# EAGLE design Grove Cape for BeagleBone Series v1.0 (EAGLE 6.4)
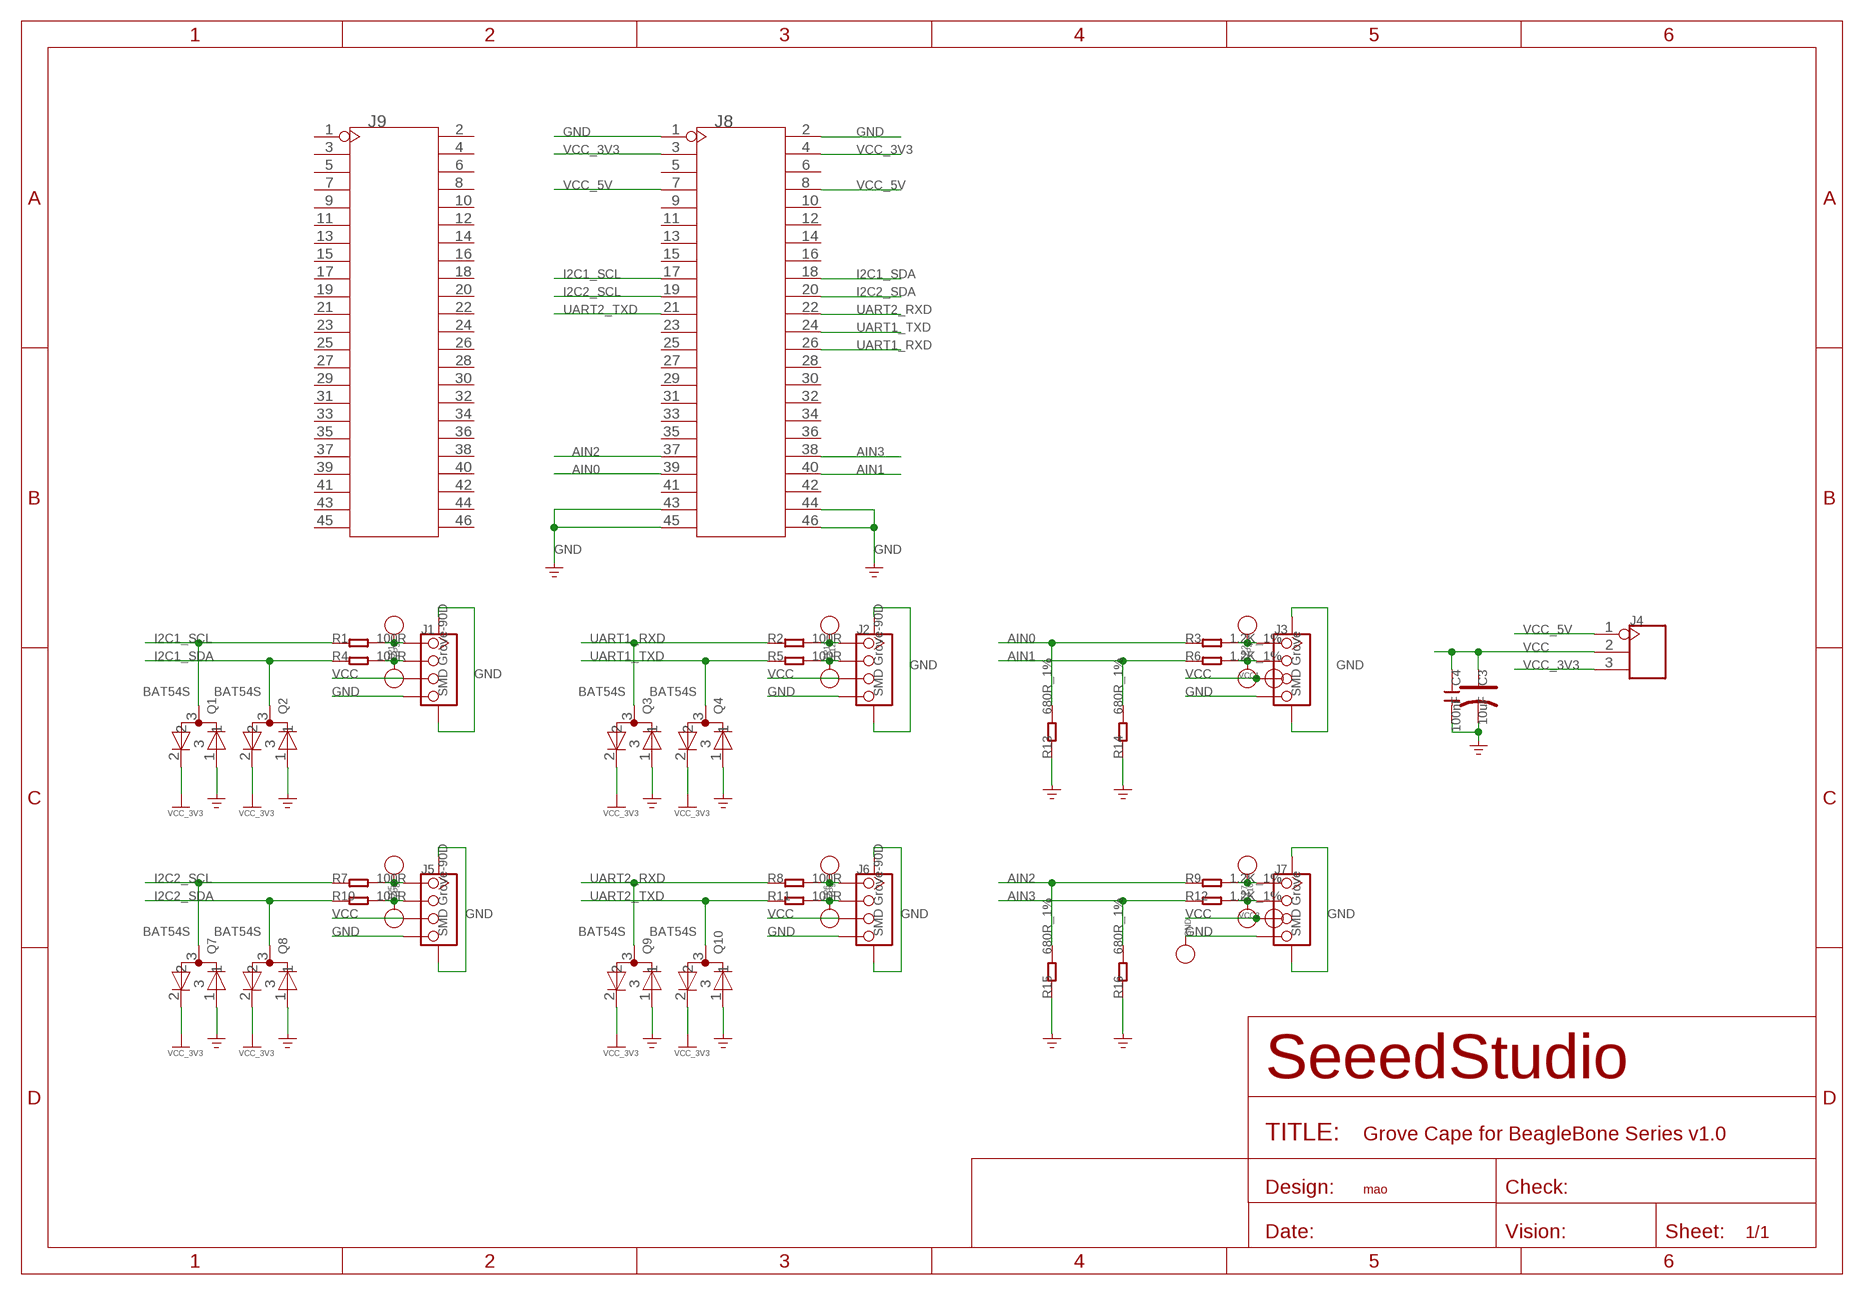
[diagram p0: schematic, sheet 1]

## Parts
C3  10uF  CAP-AVX-A  [AVX-A]
C4  100nF  C-0603  [C0603]
GND  PAD-TEST-POINT'4545'  [TP_4545]
J1  SMD Grove-90D  TWIG-4P-2.0-SMD-FEMALE-REINFORCE'DD'  [4P-SMD-2.0]
J2  SMD Grove-90D  TWIG-4P-2.0-SMD-FEMALE-REINFORCE'DD'  [4P-SMD-2.0]
J3  SMD Grove  TWIG-4P-2.0-SMD-FEMALE-REINFORCE'90D'  [4P-SMD-2.0-90D]
J4  HEADER-3P-2.54  [3P-2.54]
J5  SMD Grove-90D  TWIG-4P-2.0-SMD-FEMALE-REINFORCE'DD'  [4P-SMD-2.0]
J6  SMD Grove-90D  TWIG-4P-2.0-SMD-FEMALE-REINFORCE'DD'  [4P-SMD-2.0]
J7  SMD Grove  TWIG-4P-2.0-SMD-FEMALE-REINFORCE'90D'  [4P-SMD-2.0-90D]
J8  HEADER-2X23P  [2X23P-2.54]
J9  HEADER-2X23P  [2X23P-2.54]
Q1  BAT54S  BAV99  [SOT23]
Q2  BAT54S  BAV99  [SOT23]
Q3  BAT54S  BAV99  [SOT23]
Q4  BAT54S  BAV99  [SOT23]
Q7  BAT54S  BAV99  [SOT23]
Q8  BAT54S  BAV99  [SOT23]
Q9  BAT54S  BAV99  [SOT23]
Q10  BAT54S  BAV99  [SOT23]
R1  100R  R-0603  [R0603]
R2  100R  R-0603  [R0603]
R3  1.2K_1%  R-0603  [R0603]
R4  100R  R-0603  [R0603]
R5  100R  R-0603  [R0603]
R6  1.2K_1%  R-0603  [R0603]
R7  100R  R-0603  [R0603]
R8  100R  R-0603  [R0603]
R9  1.2K_1%  R-0603  [R0603]
R10  100R  R-0603  [R0603]
R11  100R  R-0603  [R0603]
R12  1.2K_1%  R-0603  [R0603]
R13  680R_1%  R-0603  [R0603]
R14  680R_1%  R-0603  [R0603]
R15  680R_1%  R-0603  [R0603]
R16  680R_1%  R-0603  [R0603]
TP1  PAD-TEST-POINT'4545'  [TP_4545]
TP2  PAD-TEST-POINT'4545'  [TP_4545]
TP3  PAD-TEST-POINT'4545'  [TP_4545]
TP4  PAD-TEST-POINT'4545'  [TP_4545]
TP5  PAD-TEST-POINT'4545'  [TP_4545]
TP6  PAD-TEST-POINT'4545'  [TP_4545]
TP7  PAD-TEST-POINT'4545'  [TP_4545]
TP8  PAD-TEST-POINT'4545'  [TP_4545]
TP9  PAD-TEST-POINT'4545'  [TP_4545]
TP10  PAD-TEST-POINT'4545'  [TP_4545]
TP11  PAD-TEST-POINT'4545'  [TP_4545]
TP12  PAD-TEST-POINT'4545'  [TP_4545]
VCC1  PAD-TEST-POINT'4545'  [TP_4545]
VCC2  PAD-TEST-POINT'4545'  [TP_4545]

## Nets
AIN0: J8.39 R3.1 R13.2
AIN1: J8.40 R6.1 R14.2
AIN2: J8.37 R9.1 R15.2
AIN3: J8.38 R12.1 R16.2
GND: C3.- C4.2 GND.T J1.4 J1.SS1 J1.SS2 J2.4 J2.SS1 J2.SS2 J3.4 J3.SS1 J3.SS2 J5.4 J5.SS1 J5.SS2 J6.4 J6.SS1 J6.SS2 J7.4 J7.SS1 J7.SS2 J8.1 J8.2 J8.43 J8.44 J8.45 J8.46 Q1.1 Q2.1 Q3.1 Q4.1 Q7.1 Q8.1 Q9.1 Q10.1 R13.1 R14.1 R15.1 R16.1
I2C1_SCL: J8.17 Q1.3 R1.1
I2C1_SDA: J8.18 Q2.3 R4.1
I2C2_SCL: J8.19 Q7.3 R7.1
I2C2_SDA: J8.20 Q8.3 R10.1
N$2: J7.1 R9.2 TP7.T
N$3: J7.2 R12.2 TP10.T
N$4: J1.1 R1.2 TP1.T
N$5: J1.2 R4.2 TP3.T
N$6: J2.1 R2.2 TP11.T
N$7: J2.2 R5.2 TP12.T
N$8: J5.1 R7.2 TP5.T
N$9: J5.2 R10.2 TP8.T
N$10: J6.1 R8.2 TP6.T
N$11: J6.2 R11.2 TP9.T
N$12: J3.1 R3.2 TP2.T
N$13: J3.2 R6.2 TP4.T
UART1_RXD: J8.26 Q3.3 R2.1
UART1_TXD: J8.24 Q4.3 R5.1
UART2_RXD: J8.22 Q9.3 R8.1
UART2_TXD: J8.21 Q10.3 R11.1
VCC: C3.+ C4.1 J1.3 J2.3 J3.3 J4.2 J5.3 J6.3 J7.3 VCC1.T VCC2.T
VCC_3V3: J4.3 J8.3 J8.4 Q1.2 Q2.2 Q3.2 Q4.2 Q7.2 Q8.2 Q9.2 Q10.2
VCC_5V: J4.1 J8.7 J8.8
Unconnected: J8.5 J8.6 J8.9 J8.10 J8.11 J8.12 J8.13 J8.14 J8.15 J8.16 J8.23 J8.25 J8.27 J8.28 J8.29 J8.30 J8.31 J8.32 J8.33 J8.34 J8.35 J8.36 J8.41 J8.42 J9.1 J9.2 J9.3 J9.4 J9.5 J9.6 J9.7 J9.8 J9.9 J9.10 J9.11 J9.12 J9.13 J9.14 J9.15 J9.16 J9.17 J9.18 J9.19 J9.20 J9.21 J9.22 J9.23 J9.24 J9.25 J9.26 J9.27 J9.28 J9.29 J9.30 J9.31 J9.32 J9.33 J9.34 J9.35 J9.36 J9.37 J9.38 J9.39 J9.40 J9.41 J9.42 J9.43 J9.44 J9.45 J9.46

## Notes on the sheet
- mao

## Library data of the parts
C3 = Discrete:CAP*: Electrolytic Capacitors,Tantalum Capacitors and Super Capacitors
C4 = Discrete:C*: Ceramic Capacitors
GND TP1-TP12 VCC1 VCC2 = Discrete:PAD-TEST-POINT; PARTNO: DNP
J1-J3 J5-J7 = Connector :TWIG-4P-2.0-SMD-FEMALE-REINFORCE
J4 = Connector :HEADER-3P
J8 J9 = Connector :HEADER-2X23P
Q1-Q4 Q7-Q10 = template:BAV99
R1-R16 = Discrete:R*

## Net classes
0 default: width 0.152 mm, drill 0.305 mm, clearance 0.152 mm

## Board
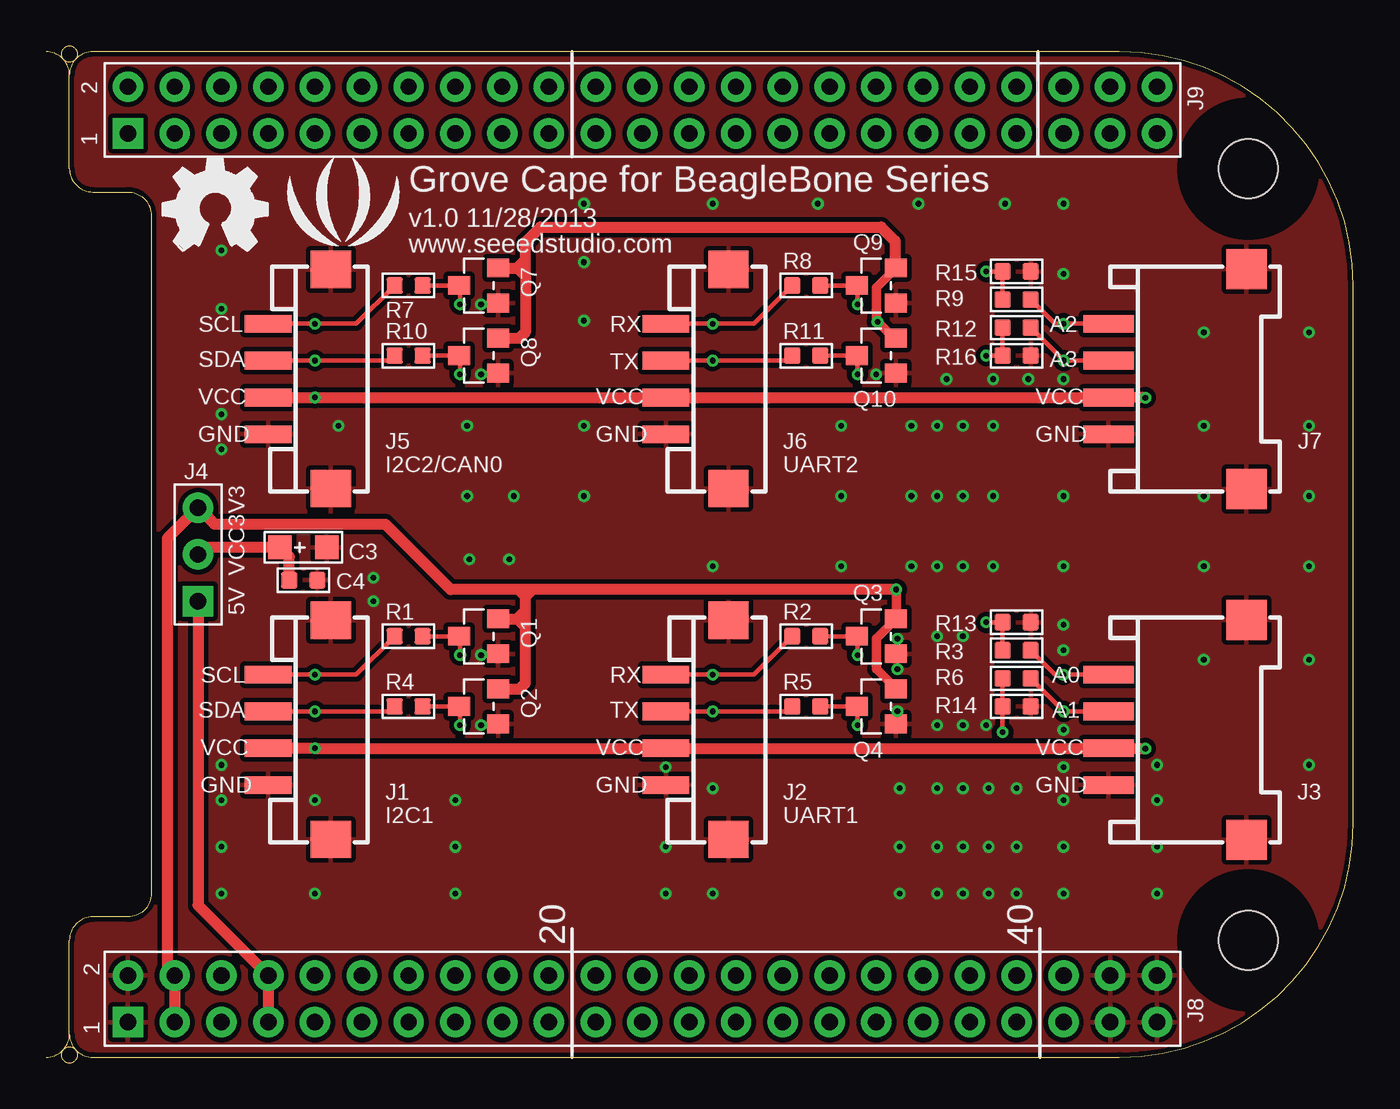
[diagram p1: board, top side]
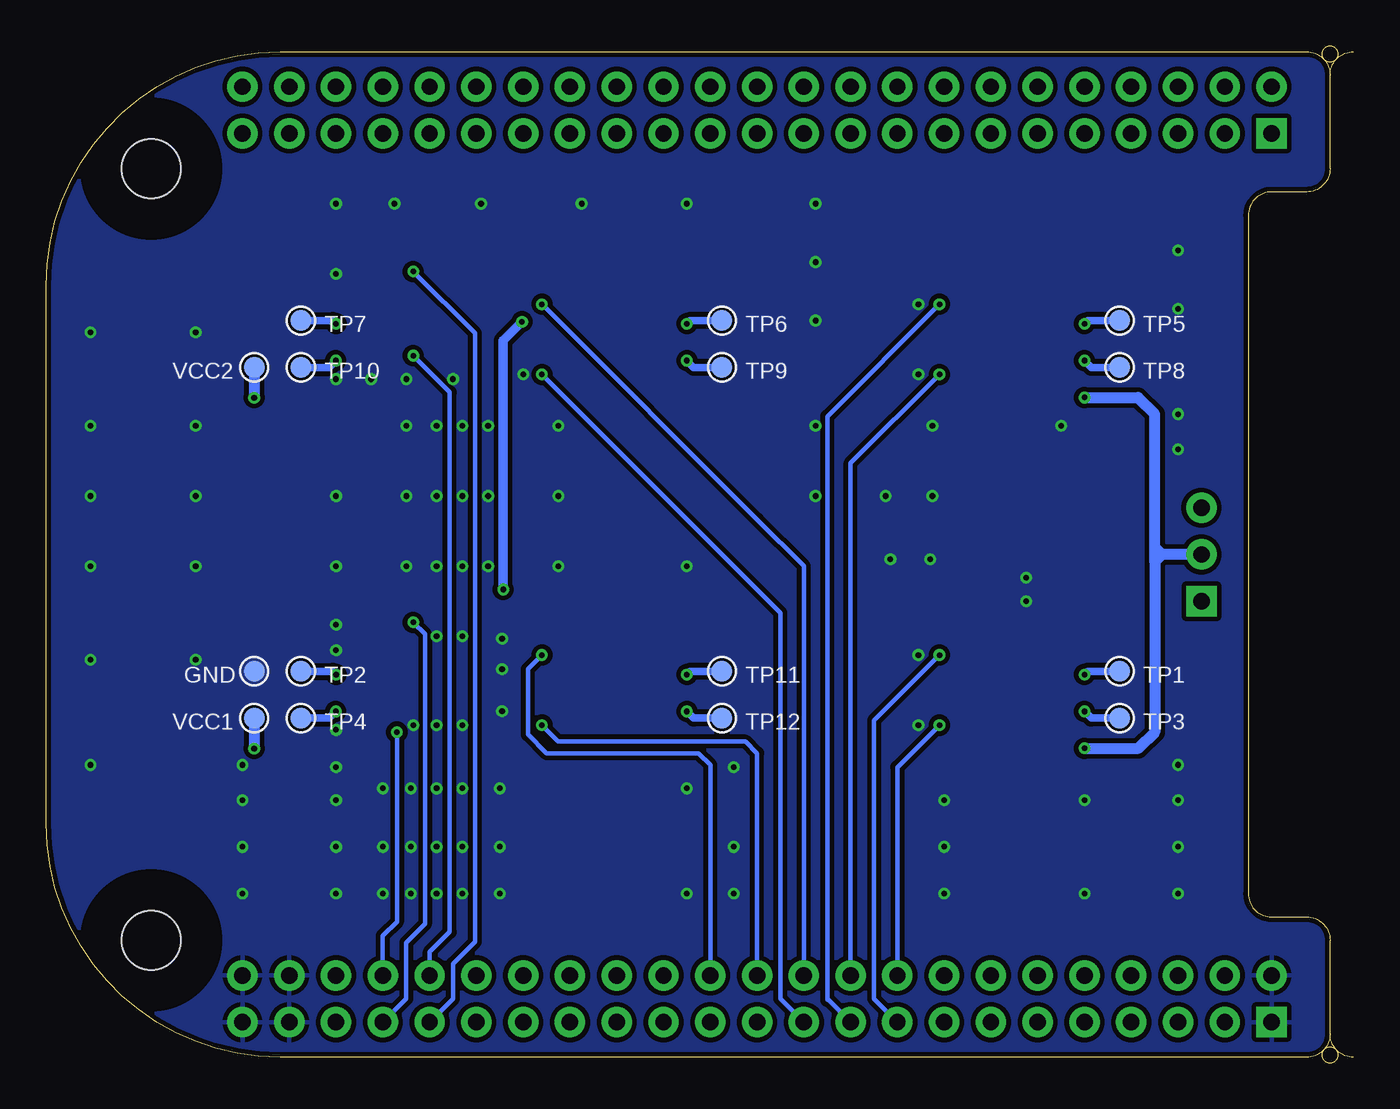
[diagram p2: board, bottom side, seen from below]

Size 70.99 x 55.22 mm. Coordinates in mm from the lower left corner, seen from the top.
Outline: 1.27,1.57 arc90 2.54,0.3 58.29,0.3 arc90 70.99,13 70.99,42.21 arc90 58.29,54.91 2.54,54.91 arc90 1.27,53.64
Outline: 1.27,53.64 1.27,48.56 arc90 2.54,47.29 4.45,47.29 arc-90 5.71,46.02 5.71,9.19 arc-90 4.45,7.92 2.54,7.92 arc90 1.27,6.65 1.27,1.57
Outline: 1.27,53.64 arc90 0,54.91
Outline: 0,0.3 arc90 1.27,1.57
Outline: circle at 1.27,0.43 radius 0.43
Outline: circle at 1.27,54.79 radius 0.43
Copper layers (1*16): Top 0.035mm / dielectric 1.1mm / Bottom 0.035mm
Design rules "SeeedStudio_rule_no_angle_090911 *": minimum track width 6mil, minimum drill 12mil, track to track 6mil, track to pad 6mil, pad to pad 6mil, via to via 6mil, smd to smd 0mil, copper to edge 3mil, drill to drill 10mil, minimum pad ring 10mil, minimum via ring 6mil, stop-mask expansion 2mil, vias tented up to drill 100mil, thermal gap 10mil

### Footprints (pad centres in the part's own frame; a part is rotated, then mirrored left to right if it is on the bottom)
AVX-A = smd 1.27 x 1.27: + -1.27,0; - 1.27,0
C0603 = smd 0.889 x 0.889: 1 -0.762,0; 2 0.762,0
TP_4545 = smd 1.143 x 1.143: T 0,0
4P-SMD-2.0 = smd 0.965 x 2.54: 1 -3,0; 2 -1,0; 3 1,0; 4 3,0 | smd 2.032 x 2.184: SS1 -5.946,3.4; SS2 5.946,3.4
4P-SMD-2.0-90D = smd 0.965 x 2.74: 1 -3,-0.1; 2 -1,-0.1; 3 1,-0.1; 4 3,-0.1 | smd 2.159 x 2.184: SS1 -5.974,7.4; SS2 5.974,7.4
3P-2.54 = drill 0.889 pad 1.651 square: 1 0,2.54 | drill 0.889 pad 1.651: 2 0,0; 3 0,-2.54
2X23P-2.54 = drill 0.889 pad 1.651 square: 1 -1.27,27.94 | drill 0.889 pad 1.651: 2 1.27,27.94; 3 -1.27,25.4; 4 1.27,25.4; 5 -1.27,22.86; 6 1.27,22.86; 7 -1.27,20.32; 8 1.27,20.32; 9 -1.27,17.78; 10 1.27,17.78; 11 -1.27,15.24; 12 1.27,15.24; 13 -1.27,12.7; 14 1.27,12.7; 15 -1.27,10.16; 16 1.27,10.16; 17 -1.27,7.62; 18 1.27,7.62; 19 -1.27,5.08; 20 1.27,5.08; 21 -1.27,2.54; 22 1.27,2.54; 23 -1.27,0; 24 1.27,0; 25 -1.27,-2.54; 26 1.27,-2.54; 27 -1.27,-5.08; 28 1.27,-5.08; 29 -1.27,-7.62; 30 1.27,-7.62; 31 -1.27,-10.16; 32 1.27,-10.16; 33 -1.27,-12.7; 34 1.27,-12.7; 35 -1.27,-15.24; 36 1.27,-15.24; 37 -1.27,-17.78; 38 1.27,-17.78; 39 -1.27,-20.32; 40 1.27,-20.32; 41 -1.27,-22.86; 42 1.27,-22.86; 43 -1.27,-25.4; 44 1.27,-25.4; 45 -1.27,-27.94; 46 1.27,-27.94
SOT23 = smd 1.016 x 1.2: 1 -0.95,-1.06; 2 0.95,-1.06; 3 0,1.06
R0603 = smd 0.889 x 0.889: 1 -0.762,0; 2 0.762,0
HOLE-3.2/7.0 = hole 3.2: 0,0

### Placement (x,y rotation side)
C3  13.97,27.99 0 top
C4  13.97,26.21 0 top
GND  59.69,21.26 0 bottom
J1  12.07,18.08 270 top
J2  33.66,18.08 270 top
J3  57.79,18.08 270 top
J4  8.25,27.61 180 top
J5  12.07,37.13 270 top
J6  33.66,37.13 270 top
J7  57.79,37.13 270 top
J8  32.38,3.48 90 top
J9  32.38,51.74 90 top
Q1  23.49,23.16 90 top
Q2  23.49,19.35 90 top
Q3  45.09,23.16 90 top
Q4  45.09,19.35 90 top
Q7  23.49,42.21 90 top
Q8  23.49,38.4 90 top
Q9  45.09,42.21 90 top
Q10  45.09,38.4 90 top
R1  19.68,23.16 180 top
R2  41.27,23.16 180 top
R3  52.71,22.4 0 top
R4  19.68,19.35 180 top
R5  41.27,19.35 180 top
R6  52.71,20.88 0 top
R7  19.68,42.21 180 top
R8  41.27,42.21 180 top
R9  52.71,41.45 0 top
R10  19.68,38.4 180 top
R11  41.27,38.4 180 top
R12  52.71,39.93 0 top
R13  52.71,23.93 180 top
R14  52.71,19.35 180 top
R15  52.71,42.98 180 top
R16  52.71,38.4 180 top
TP1  12.7,21.26 0 bottom
TP2  57.15,21.26 0 bottom
TP3  12.7,18.72 0 bottom
TP4  57.15,18.72 0 bottom
TP5  12.7,40.31 0 bottom
TP6  34.29,40.31 0 bottom
TP7  57.15,40.31 0 bottom
TP8  12.7,37.77 0 bottom
TP9  34.29,37.77 0 bottom
TP10  57.15,37.77 0 bottom
TP11  34.29,21.26 0 bottom
TP12  34.29,18.72 0 bottom
U$26  [HOLE-3.2/7.0]  65.28,48.56 0 top
U$27  [HOLE-3.2/7.0]  65.28,6.65 0 top
U$29  [LOGO_SILK]  16.13,46.02 0 top
U$33  [OSHW_FILLX200_NOTEXT]  6.35,44.12 0 top
VCC1  59.69,18.72 0 bottom
VCC2  59.69,37.77 0 bottom

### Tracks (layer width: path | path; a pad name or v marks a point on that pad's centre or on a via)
AIN0  (via drill 0.3 pad 0.64)
  Top 0.254: R3.1 R13.2 v51.05,23.93
  Bottom 0.254: J8.39 51.44,3.48 51.44,6.53 50.42,7.54 50.42,23.29 v51.05,23.93
AIN1  (via drill 0.3 pad 0.64)
  Top 0.254: R6.1 R14.2 v51.94,17.96
  Bottom 0.254: J8.40 52.71,6.91 51.94,7.67 v51.94,17.96 52.07,18.08
AIN2  (via drill 0.3 pad 0.64)
  Top 0.254: v51.05,42.98 R15.2 R9.1
  Bottom 0.254: J8.37 48.9,3.48 48.9,5.38 47.7,6.58 47.7,39.63 v51.05,42.98
AIN3  (via drill 0.3 pad 0.64)
  Top 0.254: v51.05,38.4 R16.2 R12.1
  Bottom 0.254: J8.38 50.16,6.02 49.08,7.11 49.08,36.43 v51.05,38.4
GND  (via drill 0.3 pad 0.64)
  other vias: 36.2,9.19 29.21,34.59 29.21,30.78 9.52,35.23 9.52,33.32 23.62,41.2 23.62,37.39 55.24,16.05 55.24,14.27 33.66,16.05 22.99,27.36 22.86,30.78 25.15,27.36 23.62,22.15 25.4,30.78 9.52,16.18 9.52,14.27 17.78,26.34 17.78,25.07 14.61,9.19 55.24,26.97 62.87,26.97 62.87,39.67 68.58,39.67 68.58,34.59 62.87,21.89 68.58,26.97 68.58,21.89 68.58,16.18 43.18,34.59 23.62,18.34 22.23,9.19 46.35,11.73 22.86,34.59 33.66,11.73 33.66,9.19 46.35,14.91 9.52,9.19 22.23,14.27 22.23,11.73 29.21,43.48 41.91,46.66 47.37,46.66 55.24,46.66 55.24,42.85 46.35,9.19 55.24,9.19 55.24,11.73 52.71,9.19 15.88,34.59 43.18,30.78 36.2,14.91 36.2,26.97 43.18,26.97 9.52,44.12 52.71,11.73 52.71,14.91 14.61,14.27 9.52,11.73 62.87,30.78 68.58,30.78 29.21,40.31 29.21,46.66 9.52,40.94 36.2,46.66 52.07,46.66 51.44,34.59 51.44,30.78 51.44,26.97 60.32,16.18 60.32,14.27 60.32,11.73 60.32,9.19 55.24,30.78 62.87,34.59 46.23,23.04 46.23,21.39 46.23,19.1 45.09,37.39 48.9,37.13 55.24,23.8 55.24,22.4 55.24,18.08 55.24,37.13 53.34,37.13 51.44,37.13 46.99,34.59 46.99,30.78 46.99,26.97 48.39,34.59 48.39,30.78 48.39,26.97 48.39,23.16 48.39,18.34 48.39,14.91 48.39,11.73 48.39,9.19 49.78,23.16 49.78,18.34 49.78,14.91 49.78,11.73 49.78,9.19 51.05,18.34 51.18,14.91 51.18,11.73 51.18,9.19 49.78,34.59 49.78,30.78 49.78,26.97
  pour Top (isolate 0.254): 1.27,54.91 71.12,54.91 71.12,0.3 1.27,0.3
  pour Bottom (isolate 0.254): 1.27,54.91 71.12,54.91 71.12,0.3 1.27,0.3
I2C1_SCL  (via drill 0.3 pad 0.64)
  Top 0.254: R1.1 Q1.3 22.48,23.12 v22.48,22.15
  Bottom 0.254: J8.17 26.04,3.48 26.04,18.59 v22.48,22.15
I2C1_SDA  (via drill 0.3 pad 0.64)
  Top 0.254: R4.1 Q2.3 22.48,19.31 v22.48,18.34
  Bottom 0.254: J8.18 24.77,16.05 v22.48,18.34
I2C2_SCL  (via drill 0.3 pad 0.64)
  Top 0.254: v22.48,41.2 22.48,42.17 Q7.3 R7.1
  Bottom 0.254: J8.19 28.51,3.42 28.58,3.42 28.58,35.1 v22.48,41.2
I2C2_SDA  (via drill 0.3 pad 0.64)
  Top 0.203: 20.32,38.28 R10.1
  Top 0.254: R10.1 Q8.3 22.48,38.36 v22.48,37.39
  Bottom 0.254: J8.20 27.3,32.56 v22.48,37.39
N$2  (via drill 0.3 pad 0.64)
  Top 0.254: J7.1 55.5,40.13 v55.24,40.13 54.79,40.13 R9.2
  Bottom 0.406: TP7.T 55.42,40.31 v55.24,40.13
N$3  (via drill 0.3 pad 0.64)
  Top 0.254: J7.2 55.5,38.13 v55.26,38.13 R12.2
  Bottom 0.406: TP10.T 55.63,37.77 v55.26,38.13
N$4  (via drill 0.3 pad 0.64)
  Top 0.254: J1.1 v14.61,21.08 16.84,21.08 R1.2
  Bottom 0.406: TP1.T 14.43,21.26 v14.61,21.08
N$5  (via drill 0.3 pad 0.64)
  Top 0.254: J1.2 v14.61,19.08 14.86,19.08 18.65,19.08 R4.2
  Bottom 0.406: TP3.T 14.24,18.72 v14.61,19.08
N$6  (via drill 0.3 pad 0.64)
  Top 0.254: J2.1 v36.2,21.08 38.43,21.08 R2.2
  Bottom 0.406: TP11.T 35.81,21.26 35.89,21.26 36.02,21.26 v36.2,21.08
N$7  (via drill 0.3 pad 0.64)
  Top 0.254: J2.2 v36.2,19.08 40.24,19.08 R5.2
  Bottom 0.406: TP12.T 35.83,18.72 v36.2,19.08
N$8  (via drill 0.3 pad 0.64)
  Top 0.254: J5.1 v14.61,40.13 16.84,40.13 R7.2
  Bottom 0.406: TP5.T 14.43,40.31 v14.61,40.13
N$9  (via drill 0.3 pad 0.64)
  Top 0.254: J5.2 v14.61,38.13 14.86,38.13 18.65,38.13 R10.2
  Bottom 0.406: TP8.T 14.24,37.77 v14.61,38.13
N$10  (via drill 0.3 pad 0.64)
  Top 0.254: J6.1 v36.2,40.13 38.43,40.13 R8.2
  Bottom 0.406: TP6.T 35.81,40.31 35.89,40.31 36.02,40.31 v36.2,40.13
N$11  (via drill 0.3 pad 0.64)
  Top 0.254: J6.2 35.18,38.13 v36.2,38.13 40.24,38.13 R11.2
  Bottom 0.406: TP9.T 35.83,37.77 v36.2,38.13
N$12  (via drill 0.3 pad 0.64)
  Top 0.254: J3.1 v55.24,21.08 54.79,21.08 R3.2
  Bottom 0.254: 57.02,21.08 56.98,21.08 56.77,21.08
  Bottom 0.406: 56.98,21.08 TP2.T 55.42,21.26 v55.24,21.08
N$13  (via drill 0.3 pad 0.64)
  Top 0.254: J3.2 55.75,19.08 v55.26,19.08 R6.2
  Bottom 0.406: TP4.T 55.63,18.72 v55.26,19.08
UART1_RXD  (via drill 0.3 pad 0.64)
  Top 0.254: R2.1 Q3.3 44.07,23.12 v44.07,22.15
  Bottom 0.254: J8.26 34.92,16.18 35.56,16.81 43.81,16.81 44.83,17.83 44.83,21.39 v44.07,22.15
UART1_TXD  (via drill 0.3 pad 0.64)
  Top 0.254: v44.07,18.34 44.07,19.31 Q4.3 R5.1
  Bottom 0.254: J8.24 32.38,16.81 33.02,17.45 43.18,17.45 v44.07,18.34
UART2_RXD  (via drill 0.3 pad 0.64)
  Top 0.254: R8.1 Q9.3 44.07,42.17 v44.07,41.2
  Bottom 0.254: J8.22 29.84,26.97 32.38,29.51 v44.07,41.2
UART2_TXD  (via drill 0.3 pad 0.64)
  Top 0.254: R11.1 Q10.3 44.07,38.36 v44.07,37.39
  Bottom 0.254: J8.21 31.12,3.48 31.12,24.43 34.92,28.24 v44.07,37.39
VCC  (via drill 0.3 pad 0.64)
  Top 0.61: J5.3 v14.61,36.13 J6.3 J7.3 v59.69,36.12 | J1.3 v14.61,17.08 J2.3 J3.3 59.67,17.08 v59.69,17.07 | C4.1 13.21,27.48 C3.+ 8.64,27.99 J4.2
  Bottom 0.61: VCC1.T v59.69,17.07 | VCC2.T v59.69,36.12 | J4.2 10.41,27.61 | 10.41,27.61 10.8,27.61 | 10.8,27.23 10.8,17.96 11.67,17.08 v14.61,17.08 | 10.8,27.61 10.8,27.99 | 10.8,27.99 10.8,35.23 11.7,36.13 v14.61,36.13 | 10.41,27.61 10.8,27.99 | 10.41,27.61 10.8,27.23 | 10.8,27.23 10.8,27.61
VCC_3V3  (via drill 0.3 pad 0.64)
  Top 0.508: Q9.2 45.09,42.1 45.09,40.31 v45.15,40.25 46.04,39.35 Q10.2 | Q4.2 46.15,20.33 45.09,21.39 45.09,23.05 Q3.2 46.16,24.13 v46.16,25.7
  Top 0.61: Q7.2 25.59,43.16 | 25.59,43.16 26.04,42.72 | 26.04,42.72 26.04,39.67 25.72,39.35 Q8.2 | Q2.2 25.72,20.3 26.04,20.62 26.04,23.67 | 26.04,23.67 26.04,24.18 | 26.04,24.18 26.04,24.56 | 26.04,24.56 26.04,25.32 | 26.04,25.32 26.04,25.7 | Q1.2 25.59,24.11 | 25.59,24.11 25.97,24.11 26.04,24.18 | 26.04,42.72 26.04,43.61 | 26.04,43.61 26.04,44.58 26.85,45.39 45.34,45.39 46.1,44.63 46.1,43.21 Q9.2 | v46.16,25.7 26.42,25.7 | 26.42,25.7 26.04,25.7 | 26.04,25.7 25.65,25.7 | 25.65,25.7 21.97,25.7 18.41,29.26 9.14,29.26 J4.3 6.6,28.5 6.6,5.13 J8.4 J8.3 | 25.59,24.11 26.04,24.56 | 25.59,24.11 | 25.59,24.11 26.04,23.67 | 26.04,25.32 25.65,25.7 | 26.04,25.32 26.42,25.7 | 25.59,43.16 26.04,43.61
  Bottom 0.508: v46.16,25.7 46.16,39.23 v45.15,40.25
VCC_5V
  Top 0.61: J4.1 8.25,8.56 J8.8 J8.7

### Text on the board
tPlace: 2 | 1 | Grove Cape for BeagleBone Series | v1.0 11/28/2013 | www.seeedstudio.com | SCL | RX | A2 | SDA | TX | A3 | VCC | VCC | VCC | GND | GND | GND | I2C2/CAN0 | UART2 | 3V3 | VCC | 5V | SCL | RX | A0 | SDA | TX | A1 | VCC | VCC | VCC | GND | GND | GND | I2C1 | UART1 | 20 | 40 | 2 | 1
